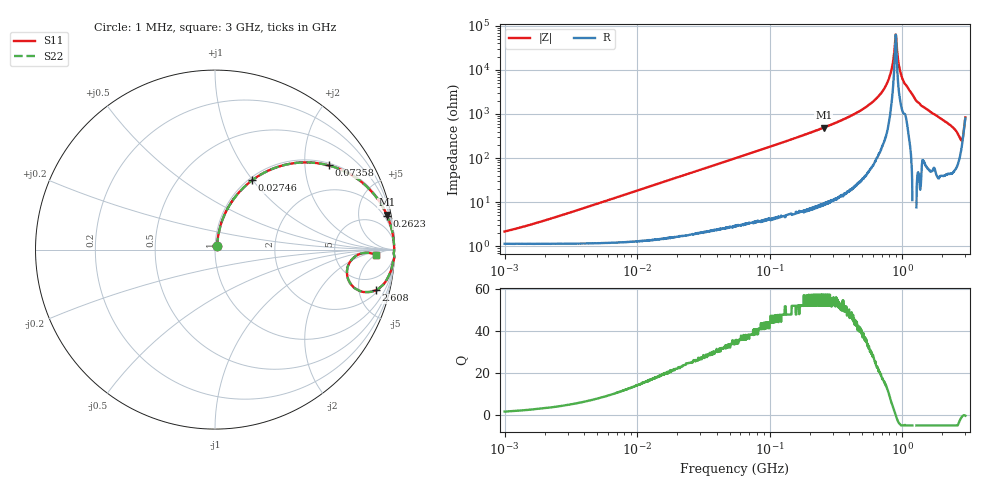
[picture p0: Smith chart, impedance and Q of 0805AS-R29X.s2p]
!s-Parameter Generated by FASTRON Sdn. Bhd.
!FASTRON P/N : 0805AS-R29X
!Keysight Technologies: E4991B_MY54100416_A.01.15
!Date: Mon Jun 15 12:53:41 2026
!Version  :Rev01  Mon Jun 15 12:53:41 2026
!Data & Calibration Information:
!Freq  S11  S21  S12  S22
!PortZ  Port1:50+j0  Port2:50+j0
!When reading reference impedance value at option line is always used.
! Remarks : This data is being provided solely for informational purposes.
# Hz S dB R 50
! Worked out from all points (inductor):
!   1601 points, 1 MHz to 3 GHz, reference 50 ohm
!   read as one part in series: L = 292 nH near 1.869 MHz
!   highest Q = 57.3 at 255.8 MHz (marker M1), where L = 304 nH
!   self-resonance near 893.7 MHz
!   S11 on the Smith chart (normalised r, x): 1 MHz: 1.02, +0.04; 27.46 MHz: 1.04, +0.99; 73.58 MHz: 1.07, +2.65; 262.3 MHz: 1, +10; 2.608 GHz: 2.34, -7.36; 3 GHz: 17, -5
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1000000  -33.40 57.1  -0.10 -1.0  -0.10 -1.0  -33.40 57.1
3804036  -23.10 76.6  -0.12 -4.0  -0.12 -4.0  -23.10 76.6
1.447069e7  -12.00 72.3  -0.41 -14.6  -0.41 -14.6  -12.00 72.3
2.745737e7  -7.15 61.8  -1.09 -26.0  -1.09 -26.0  -7.15 61.8
5.504702e7  -3.17 44.4  -3.10 -43.9  -3.10 -43.9  -3.17 44.4
7.358334e7  -2.06 36.5  -4.51 -52.0  -4.51 -52.0  -2.06 36.5
2.083556e8  -0.32 14.3  -12.10 -74.6  -12.10 -74.6  -0.32 14.3
2.558035e8  -0.21 11.5  -14.00 -77.5  -14.00 -77.5  -0.21 11.5
2.622844e8  -0.20 11.1  -14.30 -77.8  -14.30 -77.8  -0.20 11.1
5.500551e8  -0.04 3.7  -23.80 -84.6  -23.80 -84.6  -0.04 3.7
6.889699e8  -0.02 2.0  -29.30 -85.0  -29.30 -85.0  -0.02 2.0
7.925923e8  -0.01 0.9  -35.90 -83.5  -35.90 -83.5  -0.01 0.9
8.332625e8  -0.02 0.5  -40.50 -79.1  -40.50 -79.1  -0.02 0.5
8.71647e8  -0.01 0.2  -48.10 -64.5  -48.10 -64.5  -0.01 0.2
8.982141e8  -0.01 -0.0  -55.80 16.6  -55.80 16.6  -0.01 -0.0
9.209708e8  -0.01 -0.2  -47.20 67.3  -47.20 67.3  -0.01 -0.2
9.633956e8  -0.02 -0.6  -39.70 76.7  -39.70 76.7  -0.02 -0.6
1.007775e9  -0.03 -0.9  -35.80 78.5  -35.80 78.5  -0.03 -0.9
1.255985e9  -0.00 -2.7  -26.60 88.5  -26.60 88.5  -0.00 -2.7
2.607784e9  -0.67 -14.1  -12.10 65.6  -12.10 65.6  -0.67 -14.1
2.797026e9  -2.23 -13.8  -10.20 36.6  -10.20 36.6  -2.23 -13.8
3e9  -0.94 -2.0  -19.40 16.8  -19.40 16.8  -0.94 -2.0
